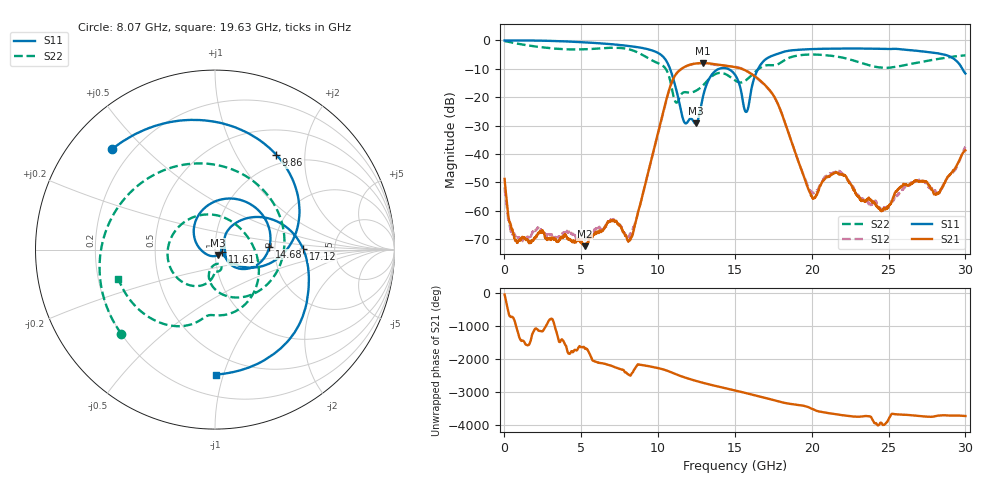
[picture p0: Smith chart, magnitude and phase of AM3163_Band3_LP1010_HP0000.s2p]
!Agilent Technologies,E8364B,MY43040894,A.07.50.67
!Agilent E8364B: A.07.50.67
!Date: Thursday, August 20, 2020 12:12:41
!Correction: S11(Full 2 Port(1,2))
!S21(Full 2 Port(1,2))
!S12(Full 2 Port(1,2))
!S22(Full 2 Port(1,2))
!S2P File: Measurements: S11, S21, S12, S22:
# Hz S  dB  R 50
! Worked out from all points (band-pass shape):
!   3201 points, 10 MHz to 30 GHz, reference 50 ohm
!   highest |S21| = -7.96 dB at 12.92 GHz (marker M1); lowest = -72.5 dB at 5.211 GHz (marker M2)
!   |S21| within 3 dB of the highest: 11.31 GHz to 15.83 GHz (4.523 GHz wide, 33.3 % of centre)
!   lowest |S11| = -29.2 dB at 12.44 GHz (marker M3), VSWR 1.07, Z = 51.7 - j3.08 ohm
!   |S11| at or under -10 dB: 10.78 GHz to 13.96 GHz (3.182 GHz wide, 25.7 % of centre); 14.55 GHz to 16.51 GHz (1.961 GHz wide, 12.6 % of centre); 29.8 GHz to end of sweep
!   |S22| runs from -21.9 to -0.3 dB; largest |S21 - S12| = 0.012
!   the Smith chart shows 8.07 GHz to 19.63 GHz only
!   S11 on the Smith chart (normalised r, x): 8.07 GHz: 0.13, +0.40; 9.86 GHz: 0.85, +1.48; 11.61 GHz: 1.08, -0.03; 14.68 GHz: 1.87, +0.07; 17.12 GHz: 2.93, +0.02; 19.63 GHz: 0.35, -0.94
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1e7  -0.02 -1.9  -48.75 -33.2  -51.77 -119.3  -0.25 -5.9
7.691219e8  -0.00 -21.0  -70.58 69.0  -69.61 23.5  -1.05 -60.4
2.456059e9  -0.08 -67.3  -67.13 -69.2  -67.13 -176.2  -2.43 -166.4
5.014581e9  -0.60 -135.6  -70.77 167.3  -70.34 -112.9  -3.16 57.6
5.211391e9  -0.67 -140.9  -72.46 149.2  -70.05 -92.6  -3.12 46.7
6.485966e9  -1.12 -175.7  -66.29 28.6  -65.93 -156.0  -2.69 -28.0
8.069812e9  -1.93 135.6  -70.57 59.7  -69.07 -41.2  -3.08 -138.2
9.128834e9  -2.82 94.8  -51.43 -26.1  -51.56 -25.3  -5.54 124.2
9.859841e9  -4.03 57.1  -35.61 -89.5  -35.63 -90.3  -7.67 36.0
1.000979e10  -4.43 47.6  -32.33 -105.4  -32.38 -106.1  -8.03 15.7
1.161238e10  -27.49 -21.2  -9.67 -9.8  -9.71 -9.8  -18.41 -76.6
1.243711e10  -29.24 -59.6  -8.12 -129.8  -8.17 -129.8  -17.79 -90.8
1.292444e10  -19.70 164.7  -7.96 167.9  -8.03 167.6  -15.83 -96.1
1.467698e10  -10.35 3.1  -9.09 -27.0  -9.07 -25.3  -12.80 137.4
1.5005e10  -12.07 -20.1  -9.37 -62.5  -9.25 -61.3  -14.08 97.8
1.574538e10  -25.16 8.1  -10.72 -146.1  -10.68 -146.5  -13.90 14.4
1.712304e10  -6.17 0.3  -16.63 53.7  -16.80 55.2  -8.71 -78.4
1.962533e10  -3.14 -89.6  -50.15 174.1  -49.47 174.0  -5.00 -163.0
2.000958e10  -3.04 -99.8  -54.92 98.6  -53.55 103.7  -4.95 -176.9
2.230569e10  -2.83 -153.3  -48.68 -110.2  -48.92 -114.1  -6.43 94.5
2.500479e10  -3.00 144.5  -58.36 149.4  -58.41 -81.8  -9.60 -53.5
3e10  -11.65 -28.3  -38.73 -118.1  -37.42 -118.6  -5.24 109.5
